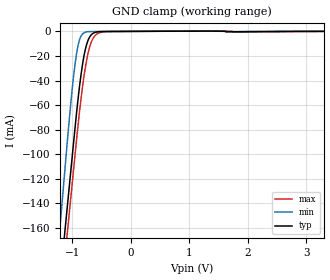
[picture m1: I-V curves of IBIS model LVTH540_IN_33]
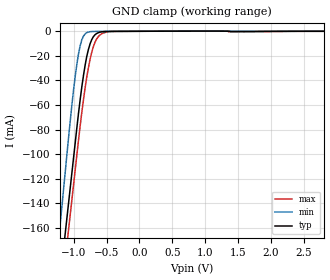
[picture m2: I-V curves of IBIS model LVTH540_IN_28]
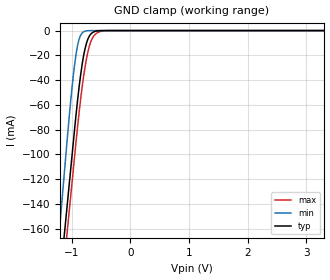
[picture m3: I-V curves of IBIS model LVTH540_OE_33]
| TEXAS INSTRUMENTS INCORPORATED
| Standard Linear and Logic Group
| IBIS Model of SN74LVTH540
| 3.3-V ABT OCTAL BUFFERS/DRIVERS WITH 3-STATE OUTPUTS
| This file contains package information for the following:
|  SSOP 20-pin (DB) package as [Component] LVTH540_DB
|  SOIC 20-pin (DW) package as [Component] LVTH540_DW
|  SOP 20-pin (NS) package as [Component] LVTH540_NS
|  TSSOP 20-pin (PW) package as [Component] LVTH540_PW
| This device can be powered at the following Vccs:
|  3.3 volt Vcc
|  2.8 volt Vcc
| This file provides unique models under the [Model Selector] for each Vcc.
| For operation at a specific Vcc, select the appropriate model after each
| [Model Selector] keyword.
[IBIS Ver]   3.2
[Comment char]  |_char
[File Name]   sn74lvth540.ibs
[File Rev]   1.1 | x_die
[Date]   June 21, 2002
[Source]   Data created from TI-SPICE simulations at TI-SLL.
[Notes]   The following is an IBIS list for the LVTH540_DL.
   Please contact sllibis@ti.com with questions and
   comments concerning SLL IBIS models.
[Disclaimer] Property of Texas Instruments Incorporated.  Unauthorized
   reproduction and/or distribution is strictly prohibited.
   This product is protected under copyright law.
   Created  2002, (C) Copyright  2002, Texas Instruments
   Incorporated, All Rights Reserved
   UNLESS THERE IS A SIGNED, WRITTEN AGREEMENT TO THE
   CONTRARY, TEXAS INSTRUMENTS (TI) IS PROVIDING THE IBIS
   MODELS  AND WITHOUT ANY WARRANTY, EXPRESSED OR
   IMPLIED.  TI assumes no liability for:
   1) the accuracy of the IBIS models provided to your
   company;
   2) the proper functioning of these IBIS Models in your
   design or for any resulting applications; or
   3) infringement of patents, copyrights or intellectual
   property rights resulting from your use of these IBIS
   models.
   TI provides IBIS Models as a service to our customers.
   You and your company shall not distribute, sell or give
   these models to anyone else without prior written
   permission from TI.
   TI reserves the right to make changes to our products or
   to discontinue any semiconductor product or service
   without notice, and advises our customers to obtain the
   latest version of relevant information to verify, before
   placing orders, that the information being relied on is
   current.
   Please be aware that your receipt and use of the IBIS
   information provided shall serve as acceptance of these
   terms and conditions.  If you do not accept these terms,
   you should return or destroy the IBIS models and any
   other accompanying information immediately.
| Component LVTH540_DL_DB 20-pin SSOP
[Component]   LVTH540_DB
[Manufacturer]   Texas Instruments, Inc.
[Package]
|   typ   min   max
R_pkg   4.000e-02   3.500e-02   5.100e-02
L_pkg   3.495e-09   3.035e-09   4.314e-09
C_pkg   4.200e-13   3.460e-13   5.020e-13
[Pin]   signal_name   model_name   R_pin   L_pin   C_pin
1   NOE1   LVTH540_OE   4.900e-02   4.310e-09   5.020e-13
2   A1   LVTH540_IN   4.800e-02   3.903e-09   4.870e-13
3   A2   LVTH540_IN   3.500e-02   3.189e-09   3.960e-13
4   A3   LVTH540_IN   3.500e-02   3.036e-09   3.470e-13
5   A4   LVTH540_IN   3.500e-02   3.035e-09   3.670e-13
6   A5   LVTH540_IN   3.500e-02   3.035e-09   3.670e-13
7   A6   LVTH540_IN   3.500e-02   3.036e-09   3.470e-13
8   A7   LVTH540_IN   3.500e-02   3.189e-09   3.970e-13
9   A8   LVTH540_IN   4.700e-02   3.899e-09   4.880e-13
10   GND   GND   5.100e-02   4.314e-09   5.000e-13
11   Y8   LVTH540_OUT   5.100e-02   4.314e-09   5.000e-13
12   Y7   LVTH540_OUT   4.700e-02   3.899e-09   4.880e-13
13   Y6   LVTH540_OUT   3.500e-02   3.189e-09   3.970e-13
14   Y5   LVTH540_OUT   3.500e-02   3.036e-09   3.460e-13
15   Y4   LVTH540_OUT   3.500e-02   3.035e-09   3.670e-13
16   Y3   LVTH540_OUT   3.500e-02   3.035e-09   3.670e-13
17   Y2   LVTH540_OUT   3.500e-02   3.036e-09   3.460e-13
18   Y1   LVTH540_OUT   3.500e-02   3.189e-09   3.970e-13
19   NOE2   LVTH540_OE   4.700e-02   3.899e-09   4.880e-13
20   VCC   POWER   5.100e-02   4.314e-09   5.020e-13
| Component LVTH540_DW 20-pin SOIC
[Component]   LVTH540_DW
[Manufacturer]   Texas Instruments, Inc.
[Package]
|   typ   min   max
R_pkg   3.800e-02   3.300e-02   4.500e-02
L_pkg   5.012e-09   4.110e-09   6.349e-09
C_pkg   7.170e-13   5.300e-13   8.680e-13
[Pin]   signal_name   model_name   R_pin   L_pin   C_pin
1   NOE1   LVTH540_OE   4.200e-02   6.336e-09   8.650e-13
2   A1   LVTH540_IN   4.300e-02   5.542e-09   8.670e-13
3   A2   LVTH540_IN   3.400e-02   4.714e-09   7.320e-13
4   A3   LVTH540_IN   3.400e-02   4.377e-09   5.910e-13
5   A4   LVTH540_IN   3.600e-02   4.130e-09   5.330e-13
6   A5   LVTH540_IN   3.500e-02   4.111e-09   5.300e-13
7   A6   LVTH540_IN   3.400e-02   4.284e-09   5.830e-13
8   A7   LVTH540_IN   3.400e-02   4.634e-09   7.260e-13
9   A8   LVTH540_IN   4.000e-02   5.518e-09   8.650e-13
10   GND   GND   4.300e-02   6.349e-09   8.660e-13
11   Y8   LVTH540_OUT   4.100e-02   6.281e-09   8.610e-13
12   Y7   LVTH540_OUT   4.500e-02   5.561e-09   8.680e-13
13   Y6   LVTH540_OUT   3.300e-02   4.778e-09   7.420e-13
14   Y5   LVTH540_OUT   3.500e-02   4.414e-09   5.960e-13
15   Y4   LVTH540_OUT   3.500e-02   4.110e-09   5.330e-13
16   Y3   LVTH540_OUT   3.600e-02   4.130e-09   5.330e-13
17   Y2   LVTH540_OUT   3.400e-02   4.377e-09   5.910e-13
18   Y1   LVTH540_OUT   3.400e-02   4.714e-09   7.310e-13
19   NOE2   LVTH540_OE   4.300e-02   5.569e-09   8.680e-13
20   VCC   POWER   4.200e-02   6.308e-09   8.640e-13
| Component LVTH540_NS 20-pin SOP
[Component]   LVTH540_NS
[Manufacturer]   Texas Instruments, Inc.
[Package]
|   typ   min   max
R_pkg   4.400e-02   2.900e-02   5.800e-02
L_pkg   3.666e-09   2.317e-09   5.115e-09
C_pkg   5.480e-13   3.160e-13   7.250e-13
[Pin]   signal_name   model_name   R_pin   L_pin   C_pin
1   NOE1   LVTH540_OE   5.800e-02   5.115e-09   7.250e-13
2   A1   LVTH540_IN   5.300e-02   4.591e-09   7.240e-13
3   A2   LVTH540_IN   4.900e-02   3.754e-09   5.720e-13
4   A3   LVTH540_IN   2.900e-02   2.549e-09   3.880e-13
5   A4   LVTH540_IN   3.100e-02   2.317e-09   3.160e-13
6   A5   LVTH540_IN   3.100e-02   2.317e-09   3.160e-13
7   A6   LVTH540_IN   2.900e-02   2.556e-09   3.990e-13
8   A7   LVTH540_IN   4.900e-02   3.754e-09   5.790e-13
9   A8   LVTH540_IN   5.300e-02   4.591e-09   7.240e-13
10   GND   GND   5.800e-02   5.115e-09   7.250e-13
11   Y8   LVTH540_OUT   5.800e-02   5.115e-09   7.250e-13
12   Y7   LVTH540_OUT   5.300e-02   4.591e-09   7.240e-13
13   Y6   LVTH540_OUT   4.900e-02   3.754e-09   5.790e-13
14   Y5   LVTH540_OUT   2.900e-02   2.557e-09   3.990e-13
15   Y4   LVTH540_OUT   3.100e-02   2.317e-09   3.160e-13
16   Y3   LVTH540_OUT   3.100e-02   2.317e-09   3.160e-13
17   Y2   LVTH540_OUT   2.900e-02   2.557e-09   3.990e-13
18   Y1   LVTH540_OUT   4.900e-02   3.754e-09   5.790e-13
19   NOE2   LVTH540_OE   5.300e-02   4.591e-09   7.240e-13
20   VCC   POWER   5.800e-02   5.115e-09   7.250e-13
| Component LVTH540_PW 20-pin TSSOP
[Component]   LVTH540_PW
[Manufacturer]   Texas Instruments, Inc.
[Package]
|   typ   min   max
R_pkg   5.000e-02   4.200e-02   6.000e-02
L_pkg   2.802e-09   2.248e-09   3.553e-09
C_pkg   3.170e-13   2.020e-13   4.430e-13
[Pin]   signal_name   model_name   R_pin   L_pin   C_pin
1   NOE1   LVTH540_OE   5.500e-02   3.461e-09   4.400e-13
2   A1   LVTH540_IN   5.500e-02   3.150e-09   4.010e-13
3   A2   LVTH540_IN   4.200e-02   2.619e-09   3.020e-13
4   A3   LVTH540_IN   4.500e-02   2.273e-09   2.020e-13
5   A4   LVTH540_IN   4.500e-02   2.248e-09   2.240e-13
6   A5   LVTH540_IN   4.500e-02   2.273e-09   2.260e-13
7   A6   LVTH540_IN   4.400e-02   2.323e-09   2.050e-13
8   A7   LVTH540_IN   4.600e-02   2.704e-09   3.070e-13
9   A8   LVTH540_IN   6.000e-02   3.265e-09   4.110e-13
10   GND   GND   5.700e-02   3.506e-09   4.360e-13
11   Y8   LVTH540_OUT   5.800e-02   3.553e-09   4.370e-13
12   Y7   LVTH540_OUT   5.800e-02   3.193e-09   4.050e-13
13   Y6   LVTH540_OUT   4.200e-02   2.704e-09   3.110e-13
14   Y5   LVTH540_OUT   4.600e-02   2.392e-09   2.100e-13
15   Y4   LVTH540_OUT   4.700e-02   2.334e-09   2.290e-13
16   Y3   LVTH540_OUT   4.700e-02   2.300e-09   2.270e-13
17   Y2   LVTH540_OUT   4.700e-02   2.349e-09   2.070e-13
18   Y1   LVTH540_OUT   4.500e-02   2.677e-09   3.060e-13
19   NOE2   LVTH540_OE   6.000e-02   3.235e-09   4.060e-13
20   VCC   POWER   5.600e-02   3.487e-09   4.430e-13
| Model LVTH540_IN
[Model Selector]   LVTH540_IN
LVTH540_IN_33   3.3 volt Vcc
LVTH540_IN_28   2.8 volt Vcc
| Model LVTH540_OE
[Model Selector]   LVTH540_OE
LVTH540_OE_33   3.3 volt Vcc
LVTH540_OE_28   2.8 volt Vcc
| Model LVTH540_OUT
[Model Selector]   LVTH540_OUT
LVTH540_OUT_33   3.3 volt Vcc
LVTH540_OUT_28   2.8 volt Vcc
| Models and submodels in the file (6): LVTH540_IN_33 (Input), LVTH540_IN_28 (Input), LVTH540_OE_33 (Input), LVTH540_OE_28 (Input), LVTH540_OUT_33 (3-state), LVTH540_OUT_28 (3-state)
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[Model]   LVTH540_IN_33
Model_type  Input
Vinl = 0.8
Vinh = 2.34
| variable   typ   min   max
C_comp   1.56pF   1.24pF   1.89pF
[Temperature Range]   40   -40   100
| Ambient temperature   25   -40   85
[Voltage range]   3.3   3   3.6
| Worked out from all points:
|   GND clamp passes 1 mA (typ) near -0.62 V on its own axis
[GND Clamp]
| LVTH540_IN_33
|   Voltage   I(typ)   I(min)   I(max)
-5.5V     -2.408A    -2.647A    -2.409A
-1.22V    -209.4mA   -166.1mA   -230.4mA
-1.125V   -163.2mA   -113.2mA   -184.6mA
-1.075V   -138.9mA   -85.42mA   -160.5mA
-975mV    -90.33mA   -36.31mA   -112.3mA
-900mV    -55.43mA   -11.64mA   -76.74mA
-825mV    -27.57mA   -2.158mA   -45.91mA
-775mV    -14.79mA   -631.5uA   -29.62mA
-725mV    -6.832mA   -223.9uA   -17.14mA
-650mV    -1.834mA   -140.7uA   -6.297mA
-405mV    -96.3uA    -83.61uA   -155.7uA
3.3V      19.45pA    12.56pA    -1.138uA
[Model]   LVTH540_IN_28
Model_type  Input
Vinl = 0.8
Vinh = 2.0
| variable   typ   min   max
C_comp   1.55pF   1.26pF   1.89pF
[Temperature Range]   40   -40   100
| Ambient temperature   25   -40   85
[Voltage range]   2.8   2.7   2.9
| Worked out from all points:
|   GND clamp passes 1 mA (typ) near -0.62 V on its own axis
[GND Clamp]
| LVTH540_IN_28
|   Voltage   I(typ)   I(min)   I(max)
-5.5V     -2.408A    -2.647A    -2.409A
-1.22V    -209.4mA   -166.1mA   -230.4mA
-1.205V   -202.1mA   -157.7mA   -223.2mA
-1.125V   -163.2mA   -113.1mA   -184.6mA
-1.075V   -138.9mA   -85.4mA    -160.5mA
-975mV    -90.32mA   -36.3mA    -112.3mA
-900mV    -55.42mA   -11.62mA   -76.73mA
-800mV    -20.4mA    -1.144mA   -37.12mA
-675mV    -2.832mA   -139.6uA   -8.888mA
-575mV    -458.4uA   -111.4uA   -2.116mA
-425mV    -91.65uA   -80.03uA   -193.6uA
2.8V      16.5pA     10.34pA    -1.624nA
[Model]   LVTH540_OE_33
Model_type  Input
Vinl = 0.8
Vinh = 2.34
| variable   typ   min   max
C_comp   1.78pF   1.38pF   2.15pF
[Temperature Range]   40   -40   100
| Ambient temperature   25   -40   85
[Voltage range]   3.3   3   3.6
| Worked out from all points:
|   GND clamp passes 1 mA (typ) near -0.62 V on its own axis
[GND Clamp]
| LVTH540_OE_33
|   Voltage   I(typ)   I(min)   I(max)
-5.5V     -2.407A    -2.647A    -2.408A
-1.22V    -209.3mA   -166mA     -230.3mA
-1.205V   -202mA     -157.5mA   -223mA
-1.125V   -163.1mA   -113mA     -184.4mA
-1.075V   -138.8mA   -85.24mA   -160.3mA
-975mV    -90.17mA   -36.12mA   -112.1mA
-900mV    -55.28mA   -11.44mA   -76.59mA
-825mV    -27.42mA   -1.98mA    -45.77mA
-775mV    -14.64mA   -464.8uA   -29.48mA
-650mV    -1.684mA   -2.076uA   -6.172mA
-395mV    -1.224uA   -43.32pA   -35.83uA
3.3V      16.15pA    8.657pA    1.272nA
